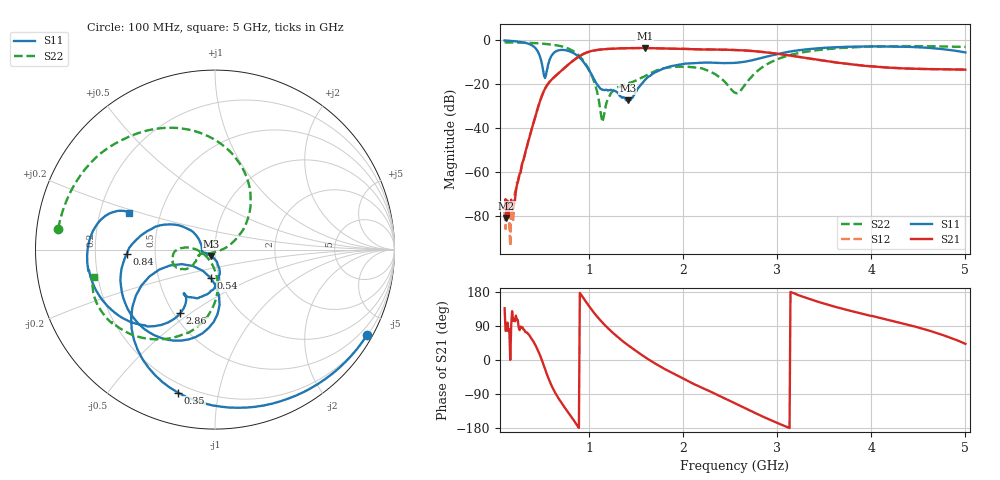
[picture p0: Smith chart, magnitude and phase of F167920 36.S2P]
!  2-Port S-parameters saved by WinCal
! VAR MeasName=S-Parameters (CALIBRATED_DATA) read from VNA (N5242A)
! VAR MeasDate=2016-11-22 9:57:11
! VAR NAME=F167920 36
! VAR FILENAME=F167920 36.S2P
! VAR DATE=2016-11-22 9:57:11
! VAR PHYS_PORTS=1,2
# Hz S DB R 50
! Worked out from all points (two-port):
!   491 points, 100 MHz to 5 GHz, reference 50 ohm
!   highest |S21| = -3.66 dB at 1.59 GHz (marker M1); lowest = -80.9 dB at 120 MHz (marker M2)
!   |S21| within 3 dB of the highest: 924.4 MHz to 3.064 GHz (2.14 GHz wide, 107 % of centre)
!   lowest |S11| = -27.5 dB at 1.41 GHz (marker M3), VSWR 1.09, Z = 47.7 - j3.4 ohm
!   |S11| at or under -10 dB: 492 MHz to 571.5 MHz (79.55 MHz wide, 15 % of centre); 938.5 MHz to 2.64 GHz (1.702 GHz wide, 95.1 % of centre)
!   |S22| runs from -37.3 to -1.1 dB; largest |S21 - S12| = 0.0015
!   S11 on the Smith chart (normalised r, x): 100 MHz: 0.22, -3.82; 350 MHz: 0.15, -0.76; 540 MHz: 0.91, -0.30; 840 MHz: 0.34, -0.02; 2.86 GHz: 0.54, -0.46; 5 GHz: 0.33, +0.18
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1e8  -0.25 -29.3  -76.78 136.6  -78.18 59.2  -1.10 172.4
1.2e8  -0.30 -35.0  -80.90 77.4  -75.20 115.3  -1.11 170.9
1.7e8  -0.47 -49.3  -72.54 90.4  -77.39 130.6  -1.14 167.0
2e8  -0.58 -58.0  -74.68 108.6  -74.58 89.1  -1.17 164.7
3.5e8  -1.69 -104.6  -46.21 68.5  -46.40 67.3  -1.33 152.2
4.5e8  -5.04 -145.3  -31.35 28.0  -31.36 28.2  -1.53 142.4
5.4e8  -15.90 -98.4  -21.38 -31.2  -21.38 -31.2  -1.85 132.3
6.6e8  -4.91 -117.9  -15.64 -95.8  -15.63 -95.7  -2.51 116.0
8.4e8  -6.16 -177.4  -9.05 -160.9  -9.04 -160.9  -5.36 79.4
9.2e8  -8.98 159.0  -6.76 169.9  -6.75 169.9  -8.49 58.5
1.05e9  -17.80 143.2  -4.81 124.8  -4.81 124.7  -18.70 24.1
1.14e9  -22.61 172.2  -4.28 98.8  -4.28 98.8  -37.30 -77.4
1.24e9  -22.83 -167.7  -4.01 74.4  -4.01 74.4  -23.62 -160.3
1.41e9  -27.51 -122.2  -3.75 39.5  -3.75 39.5  -20.04 -157.5
1.59e9  -18.32 -77.5  -3.66 8.1  -3.66 8.1  -16.52 -145.2
1.74e9  -13.89 -89.1  -3.84 -14.9  -3.83 -14.9  -13.58 -148.8
2.2e9  -10.35 -120.0  -4.36 -73.0  -4.34 -73.0  -12.96 -177.3
2.55e9  -10.41 -123.0  -4.58 -114.3  -4.57 -114.3  -23.99 -147.3
2.86e9  -7.89 -118.7  -5.54 -150.9  -5.53 -151.0  -11.85 -87.8
3.37e9  -4.03 -141.2  -8.68 158.7  -8.66 158.6  -4.96 -118.4
4.19e9  -2.95 -178.2  -12.61 105.3  -12.61 105.1  -2.87 -150.4
5e9  -5.68 156.8  -13.51 42.6  -13.52 42.6  -3.19 -167.1
